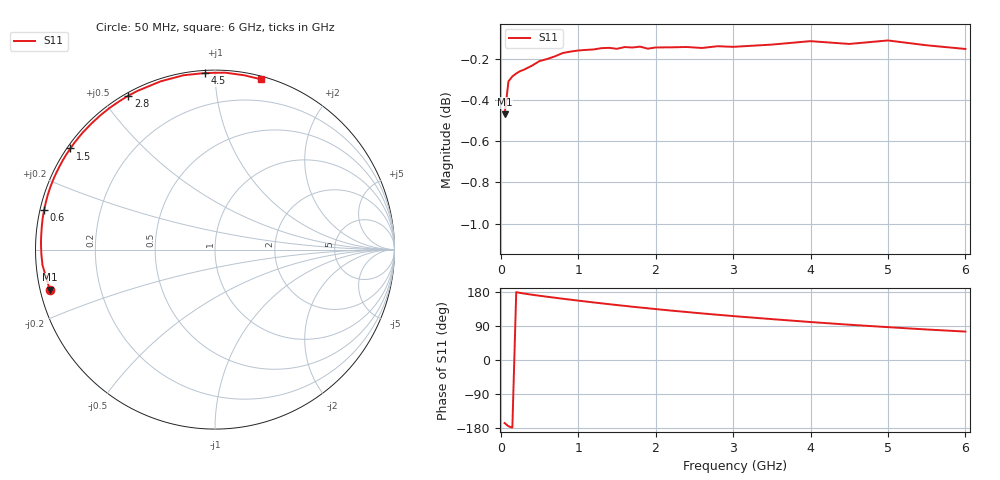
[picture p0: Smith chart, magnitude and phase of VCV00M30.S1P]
! Infineon Technologies  Discrete & RF Semiconductors
! BBY 56-03
! Si Tuning Diode in SOD323
! VR =
! S-Parameters:  June  1999
# GHz  S  MA  R  50
!  f  S11
! GHz  MAG  ANG
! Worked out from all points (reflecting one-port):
!   34 points, 50 MHz to 6 GHz, reference 50 ohm
!   lowest |S11| = -0.5 dB at 50 MHz (marker M1), VSWR 37.05, Z = 1.37 - j5.96 ohm
!   phase of S11 starts at -166 deg and turns -119 deg over the sweep
!   S11 on the Smith chart (normalised r, x): 50 MHz: 0.03, -0.12; 600 MHz: 0.01, +0.11; 1.5 GHz: 0.01, +0.32; 2.8 GHz: 0.01, +0.58; 4.5 GHz: 0.01, +0.95; 6 GHz: 0.02, +1.30
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0.05  0.9474 -166.4
0.1  0.9651 -174.9
0.15  0.9677 -178.5
0.2  0.9693 179.1
0.25  0.9706 177.1
0.3  0.9714 175.4
0.4  0.9735 172.4
0.5  0.9761 169.6
0.6  0.9772 166.9
0.8  0.9805 161.7
1  0.9819 156.7
1.2  0.9825 151.9
1.4  0.9834 147.3
1.5  0.9828 145.0
1.6  0.9838 142.9
1.8  0.984 138.5
2  0.9836 134.4
2.2  0.9836 130.4
2.4  0.9838 126.7
2.6  0.9833 122.9
2.8  0.9842 119.4
3  0.9839 115.9
3.5  0.9851 107.9
4  0.987 100.2
4.5  0.9855 93.1
5  0.9874 86.7
5.5  0.9848 80.5
6  0.9827 75.0
